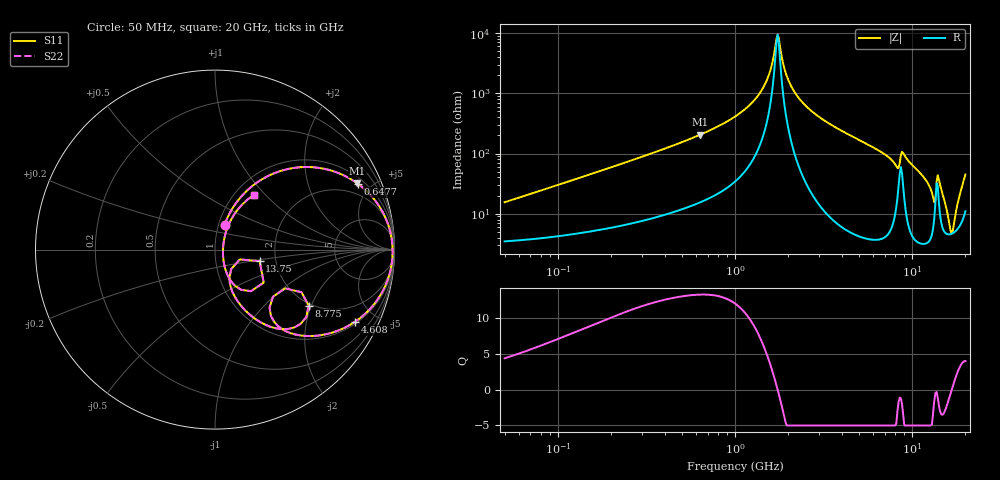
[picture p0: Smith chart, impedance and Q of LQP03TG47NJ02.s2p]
!Murata Part Number: LQP03TG47NJ02
!These Parameters are Measured in Series Mode Connection
!  o--[Z]--o
!Port1  Port2
!  o-------o
!Freq. Start=50[MHz] Stop=20[GHz], 401[Steps]
# Hz S RI R 50
!Freq.(Hz) S11(Real) S11(Imag) S21(Real) S21(Imag) S12(Real) S12(Imag) S22(Real) S22(Imag)
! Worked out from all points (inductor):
!   401 points, 50 MHz to 20 GHz, reference 50 ohm
!   read as one part in series: L = 47.8 nH near 51.52 MHz
!   highest Q = 13.2 at 638 MHz (marker M1), where L = 51.3 nH
!   self-resonance near 1.715 GHz
!   S11 on the Smith chart (normalised r, x): 50 MHz: 1.07, +0.30; 647.7 MHz: 1.32, +4.19; 4.608 GHz: 1.09, -3.82; 8.775 GHz: 1.93, -1.92; 13.75 GHz: 1.64, -0.23; 20 GHz: 1.22, +0.87
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5e7  0.0538 0.1383  0.9462 -0.1383  0.9462 -0.1383  0.0538 0.1383
1.364002e8  0.169 0.3198  0.831 -0.3198  0.831 -0.3198  0.169 0.3198
3.721004e8  0.549 0.4586  0.451 -0.4586  0.451 -0.4586  0.549 0.4586
6.380365e8  0.7921 0.3698  0.2079 -0.3698  0.2079 -0.3698  0.7921 0.3698
6.476653e8  0.7978 0.3656  0.2022 -0.3656  0.2022 -0.3656  0.7978 0.3656
1e9  0.9276 0.2208  0.0724 -0.2208  0.0724 -0.2208  0.9276 0.2208
1.432596e9  0.9807 0.0799  0.0193 -0.0799  0.0193 -0.0799  0.9807 0.0799
1.567309e9  0.9865 0.0433  0.0135 -0.0433  0.0135 -0.0433  0.9865 0.0433
1.740566e9  0.9896 -1.64e-05  0.0104 1.64e-05  0.0104 1.64e-05  0.9896 -1.64e-05
2.05233e9  0.986 -0.069  0.014 0.069  0.014 0.069  0.986 -0.069
2.728004e9  0.9536 -0.1904  0.0464 0.1904  0.0464 0.1904  0.9536 -0.1904
4.608136e9  0.7797 -0.4024  0.2203 0.4024  0.2203 0.4024  0.7797 -0.4024
7.442007e9  0.4232 -0.466  0.5768 0.466  0.5768 0.466  0.4232 -0.466
8.141811e9  0.3117 -0.3695  0.6883 0.3695  0.6883 0.3695  0.3117 -0.3695
8.774992e9  0.5219 -0.3122  0.4781 0.3122  0.4781 0.3122  0.5219 -0.3122
1.004137e10  0.3021 -0.4275  0.6979 0.4275  0.6979 0.4275  0.3021 -0.4275
1.201863e10  0.1329 -0.297  0.8671 0.297  0.8671 0.297  0.1329 -0.297
1.314879e10  0.0802 -0.1554  0.9198 0.1554  0.9198 0.1554  0.0802 -0.1554
1.375312e10  0.2486 -0.0641  0.7514 0.0641  0.7514 0.0641  0.2486 -0.0641
1.438523e10  0.146 -0.2239  0.854 0.2239  0.854 0.2239  0.146 -0.2239
1.670968e10  0.0444 -0.00347  0.9556 0.00347  0.9556 0.00347  0.0444 -0.00347
2e10  0.219 0.3063  0.781 -0.3063  0.781 -0.3063  0.219 0.3063
